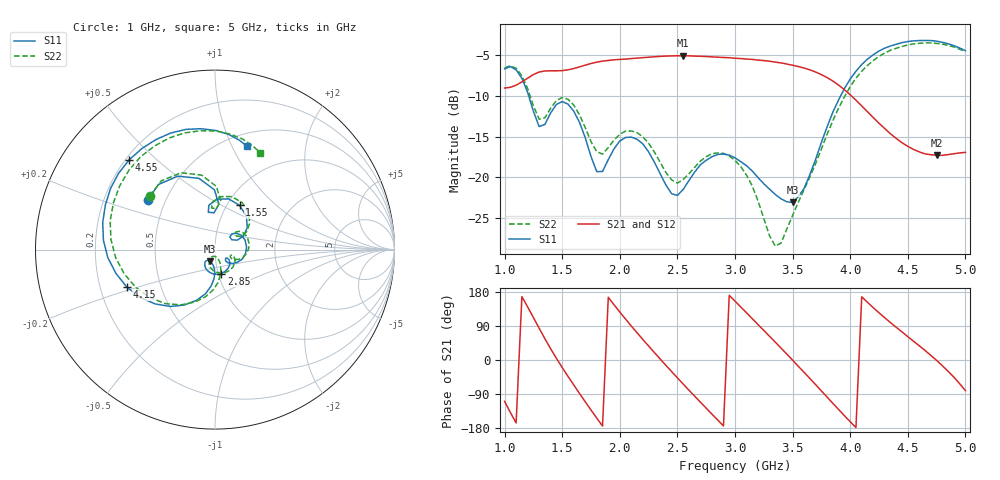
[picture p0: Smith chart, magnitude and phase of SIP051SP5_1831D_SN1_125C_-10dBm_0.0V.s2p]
# GHz  S  dB  R  50
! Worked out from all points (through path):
!   81 points, 1 GHz to 5 GHz, reference 50 ohm
!   highest |S21| = -5.03 dB at 2.55 GHz (marker M1); lowest = -17.3 dB at 4.75 GHz (marker M2)
!   lowest |S11| = -23.1 dB at 3.5 GHz (marker M3), VSWR 1.15, Z = 46.9 - j6.04 ohm
!   |S11| at or under -10 dB: 1.21 GHz to 3.916 GHz (2.706 GHz wide, 106 % of centre)
!   |S22| runs from -28.5 to -3.5 dB; largest |S21 - S12| = 0.0026
!   S11 on the Smith chart (normalised r, x): 1 GHz: 0.40, +0.28; 1.55 GHz: 1.14, +0.61; 2.85 GHz: 1.04, -0.28; 4.15 GHz: 0.31, -0.18; 4.55 GHz: 0.21, +0.41; 5 GHz: 0.63, +1.15
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1  -6.65 143.2  -9.01 -109.1  -9.01 -109.0  -6.54 140.3
1.15  -7.81 102.7  -8.26 167.2  -8.25 167.2  -7.50 100.2
1.3  -13.76 91.4  -7.04 83.8  -7.03 83.9  -12.85 87.8
1.45  -11.03 87.8  -6.89 4.2  -6.88 4.2  -10.55 83.9
1.55  -10.99 61.0  -6.77 -43.2  -6.76 -43.2  -10.38 60.0
1.7  -15.13 25.3  -6.19 -110.2  -6.19 -110.2  -13.88 29.5
1.85  -19.29 40.3  -5.70 -174.2  -5.69 -174.2  -17.14 37.5
2.05  -15.10 17.3  -5.45 107.9  -5.45 108.0  -14.30 21.4
2.35  -19.55 -45.0  -5.11 2.7  -5.10 2.8  -18.14 -26.4
2.55  -21.50 -34.5  -5.03 -63.4  -5.03 -63.5  -20.28 -18.3
2.85  -17.19 -74.9  -5.21 -158.4  -5.20 -158.3  -17.00 -55.2
3  -17.60 -101.1  -5.34 155.4  -5.33 155.2  -17.92 -85.7
3.25  -20.80 -127.9  -5.63 78.1  -5.63 78.1  -25.08 -118.6
3.35  -22.12 -127.7  -5.82 47.0  -5.82 46.9  -28.48 -101.9
3.5  -23.09 -113.9  -6.21 -0.4  -6.20 -0.3  -24.70 -70.9
3.7  -17.80 -90.5  -7.04 -65.0  -7.04 -65.2  -18.30 -74.7
3.95  -9.07 -118.8  -9.21 -147.1  -9.22 -146.8  -10.09 -111.0
4.15  -5.44 -157.1  -11.93 152.2  -11.93 152.2  -6.23 -154.2
4.35  -3.83 166.5  -14.65 98.5  -14.66 98.6  -4.36 164.8
4.55  -3.20 133.6  -16.57 49.3  -16.57 49.6  -3.57 128.8
4.75  -3.23 103.5  -17.29 -1.1  -17.30 -1.0  -3.51 96.8
5  -4.40 72.7  -16.94 -80.7  -16.95 -81.0  -4.51 64.8
